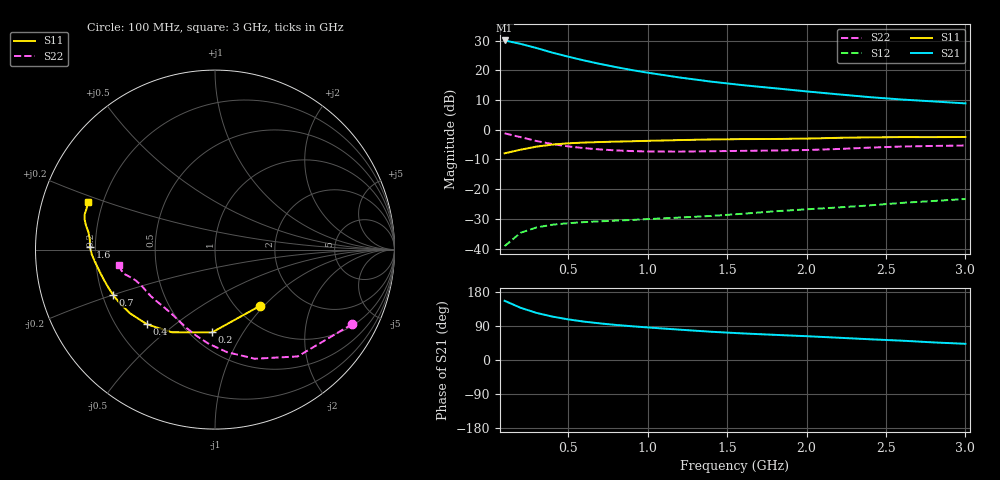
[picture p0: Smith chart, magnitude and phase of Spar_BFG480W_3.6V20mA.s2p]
! Filename: 3_620BFG480.001
! Title: BFG480W
! Bias: Vce=3.6V; Ic=20mA
! Company: NXP Semiconductors NL
! User: Quality&Reliability T&D
! Measure time: 10 Nov 1999 / 11:59:23
#  MHz  S  MA  R 50
! Freq  S11  S21  S12  S22  :
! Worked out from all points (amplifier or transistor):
!   20 points, 100 MHz to 3 GHz, reference 50 ohm
!   highest |S21| = 30.1 dB at 100 MHz (marker M1)
!   |S21| within 3 dB of that: start of sweep to 329.8 MHz
!   unconditionally stable (mu >= 1): 1.365 GHz to end of sweep
!   at 400 MHz: K = 0.39, MSG = 29.0 dB, |S12| = -32.0 dB
!   at 1.2 GHz: K = 0.94, MSG = 23.6 dB, |S12| = -29.6 dB
!   at 3 GHz: K = 1.10, MAG = 14.2 dB, |S12| = -23.3 dB
!   S11 on the Smith chart (normalised r, x): 100 MHz: 1.27, -0.95; 200 MHz: 0.63, -0.74; 400 MHz: 0.33, -0.40; 700 MHz: 0.24, -0.20; 1.6 GHz: 0.18, +0.01; 3 GHz: 0.14, +0.18
100  0.4012 -51.6  31.93 156.2  0.01096 65.7  0.87 -28.5
200  0.4614 -92.0  28 137.9  0.0184 54.3  0.7526 -52.3
300  0.5199 -117.7  23.84 124.4  0.02265 46.8  0.6473 -69.9
400  0.5628 -132.3  19.93 114.7  0.02519 42.5  0.5748 -83.4
500  0.5913 -143.0  17.04 107.2  0.0267 40.4  0.5248 -94.1
600  0.6091 -150.5  14.7 101.3  0.02784 39.6  0.4905 -102.4
700  0.6216 -156.2  12.86 96.6  0.02872 40.0  0.4664 -109.3
800  0.6315 -160.8  11.38 92.5  0.02953 41.0  0.4492 -115.0
900  0.6409 -164.6  10.14 89.1  0.03028 42.6  0.4379 -120.1
1000  0.6507 -168.1  9.156 85.9  0.03129 44.2  0.4309 -124.8
1200  0.6703 -173.7  7.603 80.1  0.03321 47.8  0.4289 -132.9
1400  0.6868 -177.7  6.468 74.5  0.03537 51.4  0.4353 -139.2
1600  0.6966 178.8  5.636 70.1  0.03855 55.3  0.4415 -144.0
1800  0.6999 175.4  5.006 66.4  0.04238 58.9  0.4475 -148.7
2000  0.7109 172.3  4.427 62.8  0.04574 62.0  0.456 -154.0
2200  0.7316 169.3  3.951 58.8  0.04922 64.1  0.4748 -158.9
2400  0.7462 166.9  3.542 54.7  0.05339 65.6  0.5004 -162.5
2600  0.7524 164.8  3.232 51.0  0.05874 66.7  0.5226 -164.9
2800  0.751 162.2  3.001 46.4  0.06325 66.7  0.5342 -167.4
3000  0.7567 159.3  2.782 42.7  0.06826 67.1  0.543 -170.8
